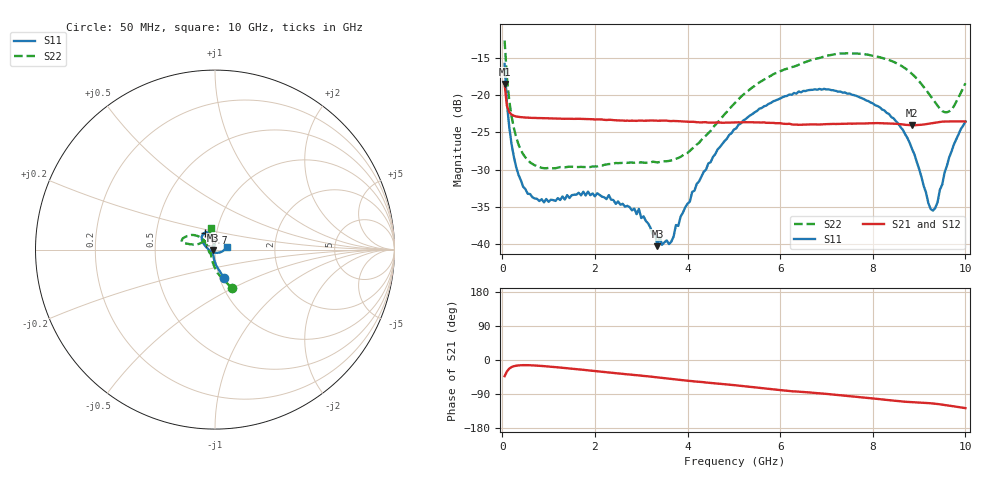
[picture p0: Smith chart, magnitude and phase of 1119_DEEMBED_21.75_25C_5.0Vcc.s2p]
!Hittite Microwave Corp.
!Digital Attenuator/PhaseShifter Rev 1.4.0
!Filename: C:\DATA\DATA\1119_DEEMBED_21.75_25C_5.0Vcc.s2p
!VNA ID: Agilent Technologies,N5224A,MY51441122,A.10.45.03
!Device type:
!2 Port Calibration.
!Temp(C): 25
!Lot Number:
!Serial Number:
!Operator:
!Misc:
!Attenuator:  21.750
# GHZ S DB R 50.0
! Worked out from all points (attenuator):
!   200 points, 50 MHz to 10 GHz, reference 50 ohm
!   highest |S21| = -18.48 dB at 50 MHz (marker M1); lowest = -24.0 dB at 8.85 GHz (marker M2)
!   lowest |S11| = -40.3 dB at 3.35 GHz (marker M3), VSWR 1.02, Z = 49.1 - j0.211 ohm
!   |S11| at or under -10 dB: start of sweep to end of sweep
!   |S22| runs from -29.8 to -12.6 dB; largest |S21 - S12| = 0.00023
!   S11 on the Smith chart (normalised r, x): 50 MHz: 1.05, -0.33; 6.7 GHz: 0.88, +0.17; 10 GHz: 1.14, +0.04
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0.05  -15.76 -72.8  -18.48 -42.8  -18.49 -42.8  -12.60 -66.5
0.1  -21.08 -85.9  -21.43 -30.0  -21.42 -30.0  -17.56 -83.4
0.2  -26.58 -98.7  -22.59 -18.7  -22.59 -18.7  -22.83 -100.1
0.45  -32.31 -116.5  -22.97 -13.6  -22.97 -13.6  -27.93 -120.8
0.9  -34.43 -133.6  -23.08 -16.2  -23.08 -16.2  -29.82 -135.0
1.75  -32.99 -141.1  -23.18 -26.0  -23.18 -26.0  -29.66 -139.7
2.95  -35.31 -138.9  -23.40 -40.6  -23.41 -40.6  -29.05 -158.7
3.3  -38.62 -164.5  -23.40 -45.3  -23.41 -45.3  -28.99 -169.1
3.35  -40.33 -167.1  -23.42 -45.9  -23.42 -46.0  -29.04 -170.7
3.4  -39.11 -174.7  -23.42 -46.5  -23.42 -46.5  -28.98 -172.1
3.65  -39.72 139.9  -23.47 -49.9  -23.48 -50.0  -28.77 178.9
3.75  -37.48 128.0  -23.46 -51.4  -23.47 -51.4  -28.55 174.8
4.45  -29.17 96.5  -23.68 -60.1  -23.69 -60.1  -25.08 147.5
5.05  -24.45 100.0  -23.65 -66.9  -23.67 -66.9  -20.84 139.5
5.85  -20.81 110.1  -23.71 -77.6  -23.72 -77.6  -17.16 144.7
6.7  -19.25 121.5  -23.91 -86.4  -23.92 -86.4  -15.18 154.5
7.5  -19.75 136.0  -23.81 -95.4  -23.82 -95.4  -14.34 163.9
8.35  -22.51 150.9  -23.79 -106.0  -23.79 -106.0  -15.23 168.1
8.85  -27.26 169.3  -24.03 -111.2  -24.03 -111.1  -17.13 167.7
9.3  -35.54 -100.5  -23.73 -114.8  -23.74 -114.8  -20.53 159.9
9.65  -28.36 -18.6  -23.52 -120.5  -23.53 -120.6  -22.16 127.1
10  -23.52 14.2  -23.54 -127.0  -23.54 -126.9  -18.37 99.5
